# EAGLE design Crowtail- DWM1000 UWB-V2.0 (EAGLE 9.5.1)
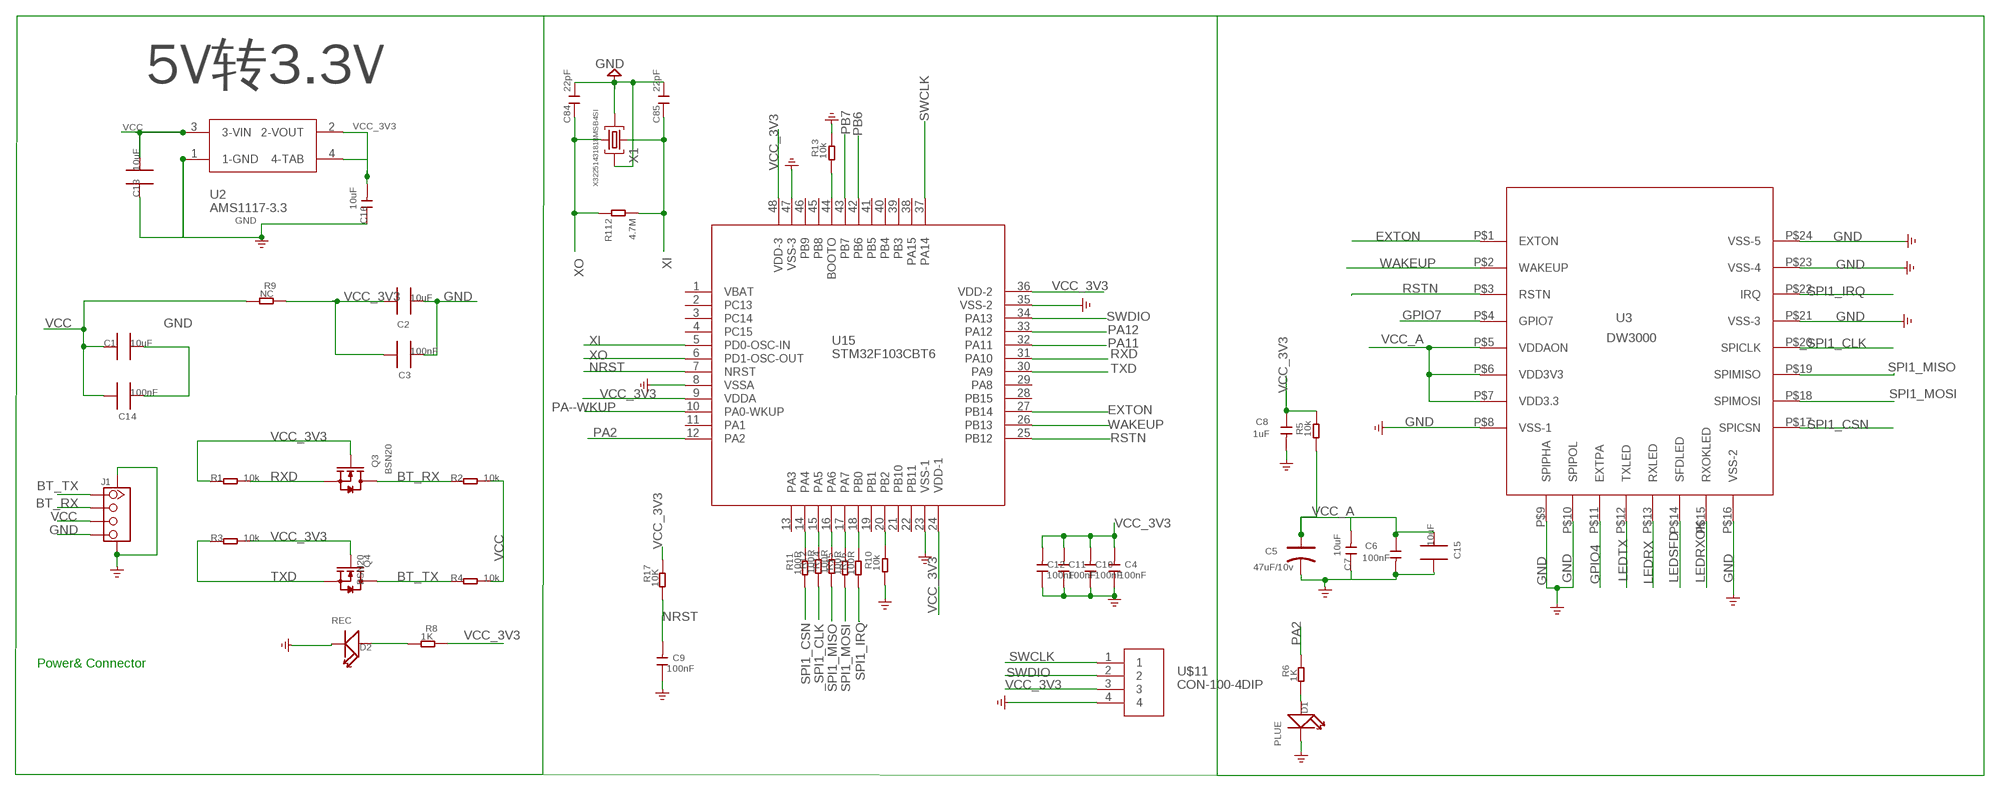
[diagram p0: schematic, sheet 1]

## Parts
C1  10uF  C0805_S  [0805_S]
C2  10uF  C0805_S  [0805_S]
C3  100nF  C0603_S  [0603_S]
C4  100nF  C-0603  [C0603]
C5  47uF/10v  CAP-AVX-B  [AVX-B]
C6  100nF  C-0603  [C0603]
C7  10uF  C-0805  [C0805]
C8  1uF  C-0603  [C0603]
C9  100nF  C-0603  [C0603]
C10  100nF  C-0603  [C0603]
C11  100nF  C-0603  [C0603]
C12  100nF  C-0603  [C0603]
C13  10uF  C0805_S  [0805_S]
C14  100nF  C0603_S  [0603_S]
C15  10uF  C0805_S  [0805_S]
C16  10uF  C-0805  [C0805]
C84  22pF  C0603  [0603]
C85  22pF  C0603  [0603]
D1  PLUE  LED'0603'  [LED-0603]
D2  REC  LED'0603'  [LED-0603]
J1  TWIG-4P-2.0-SMD-FEMALE-REINFORCE'90D'  [4P-SMD-2.0-90D]
Q3  BSN20  MOSFET-N'SOT23'  [SOT23]
Q4  BSN20  MOSFET-N'SOT23'  [SOT23]
R1  10k  R-0603  [R0603]
R2  10k  R-0603  [R0603]
R3  10k  R-0603  [R0603]
R4  10k  R-0603  [R0603]
R5  10k  R-0603  [R0603]
R6  1K  R-0603  [R0603]
R8  1K  R-0603  [R0603]
R9  NC  R-0603  [R0603]
R10  10k  R-0603  [R0603]
R11  100R  R-0603  [R0603]
R12  100R  R-0603  [R0603]
R13  10k  R-0603  [R0603]
R14  100R  R-0603  [R0603]
R15  100R  R-0603  [R0603]
R16  100R  R-0603  [R0603]
R17  10K  R-0603  [R0603]
R112  4.7M  R0603  [R0603]
U2  AMS1117-3.3  [AMS1117-3.3-SOT223]
U3  DW3000  DW1000  [DW1000]
U15  STM32F103CBT6  [LQFO48]
U$11  CON-100-4DIP  [DIP-2.54-4]
X1  X32251431818MSB4SI  CRYSTAL-3.2-2.5  [CRYSTAL-3.2-2.5]

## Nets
_SPI1_CLK: R12.1 U3.P$20(SPICLK)
BT_RX: J1.2 Q3.3(D) R2.1
BT_TX: J1.1 Q4.3(D) R4.1
EXTON: U3.P$1(EXTON) U15.27(PB14)
GND: C1.2 C2.2 C3.2 C4.1 C5.- C6.2 C7.1 C8.2 C9.1 C10.1 C11.1 C12.1 C13.1 C14.2 C15.1 C16.1 C84.1 C85.1 D1.- D2.- J1.4 J1.SS1 J1.SS2 R10.1 R13.2 U2.1(1-GND) U3.P$8(VSS-1) U3.P$9(SPIPHA) U3.P$10(SPIPOL) U3.P$16(VSS-2) U3.P$21(VSS-3) U3.P$23(VSS-4) U3.P$24(VSS-5) U15.8(VSSA) U15.23(VSS-1) U15.35(VSS-2) U15.47(VSS-3) U$11.4 X1.2(GND) X1.4(GND)
GPIO4: U3.P$11(EXTPA)
GPIO7: U3.P$4(GPIO7)
LEDRX: U3.P$13(RXLED)
LEDRXOK: U3.P$15(RXOKLED)
LEDSFD: U3.P$14(SFDLED)
LEDTX: U3.P$12(TXLED)
N$2: R10.2 U15.20(PB2)
N$3: R13.1 U15.44(BOOTO)
N$4: D1.+ R6.1
N$5: D2.+ R8.1
N$7: R11.2 U15.14(PA4)
N$8: R12.2 U15.15(PA5)
N$9: R14.2 U15.16(PA6)
N$10: R15.2 U15.17(PA7)
N$12: R16.2 U15.18(PB0)
NRST: C9.2 R17.1 U15.7(NRST)
PA2: R6.2 U15.12(PA2)
PA11: U15.32(PA11)
PA12: U15.33(PA12)
PA--WKUP: U15.10(PA0-WKUP)
PB6: U15.42(PB6)
PB7: U15.43(PB7)
RSTN: U3.P$3(RSTN) U15.25(PB12)
RXD: Q3.2(S) R1.2 U15.31(PA10)
SPI1_CSN: R11.1 U3.P$17(SPICSN)
SPI1_IRQ: R16.1 U3.P$22(IRQ)
SPI1_MISO: R14.1 U3.P$19(SPIMISO)
SPI1_MOSI: R15.1 U3.P$18(SPIMOSI)
SWCLK: U15.37(PA14) U$11.1
SWDIO: U15.34(PA13) U$11.2
TXD: Q4.2(S) R3.1 U15.30(PA9)
VCC: C1.1 C13.2 C14.1 J1.3 R2.2 R4.2 R9.1 U2.3(3-VIN)
VCC_3V3: C2.1 C3.1 C4.2 C8.1 C10.2 C11.2 C12.2 C16.2 Q3.1(G) Q4.1(G) R1.1 R3.2 R5.2 R8.2 R9.2 R17.2 U2.2(2-VOUT) U2.4(4-TAB) U15.9(VDDA) U15.24(VDD-1) U15.36(VDD-2) U15.48(VDD-3) U$11.3
VCC_A: C5.+ C6.1 C7.2 C15.2 R5.1 U3.P$5(VDDAON) U3.P$6(VDD3V3) U3.P$7(VDD3.3)
WAKEUP: U3.P$2(WAKEUP) U15.26(PB13)
XI: C85.2 R112.1 U15.5(PD0-OSC-IN) X1.3(C2)
XO: C84.2 R112.2 U15.6(PD1-OSC-OUT) X1.1(C1)
Unconnected: U15.1(VBAT) U15.2(PC13) U15.3(PC14) U15.4(PC15) U15.11(PA1) U15.13(PA3) U15.19(PB1) U15.21(PB10) U15.22(PB11) U15.28(PB15) U15.29(PA8) U15.38(PA15) U15.39(PB3) U15.40(PB4) U15.41(PB5) U15.45(PB8) U15.46(PB9)

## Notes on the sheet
- 5V转3.3V
- Power& Connector

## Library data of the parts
C1 C2 C13 C15 = CPT_SMD:C0805
C3 C14 = CPT_SMD:C0603
C4 C6 C8-C12 = discrete:C*: Ceramic Capacitors
C5 = discrete:CAP*: Electrolytic Capacitors,Tantalum Capacitors and Super Capacitors
C7 C16 = Discrete:C*: Ceramic Capacitors
C84 C85 = cooper:C0603
D1 D2 = discrete:LED*
J1 = Connector:TWIG-4P-2.0-SMD-FEMALE-REINFORCE
Q3 Q4 = discrete:MOSFET-N: IRLL014: http://www.vishay.com/docs/91319/sihll014.pdf
R1-R6 R8-R17 = discrete:R*
R112 = cooper:R0603
U2 = Crowtail- LoRA module-V1.0:AMS1117-3.3
U3 = DW1000:DW1000
U15 = DFN8:STM32F103CBT6
U$11 = DW1000:CON-100-4DIP
X1 = SmartPrj:CRYSTAL-3.2-2.5

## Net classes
0 default: width 0.152 mm, drill 0.305 mm, clearance 0.203 mm

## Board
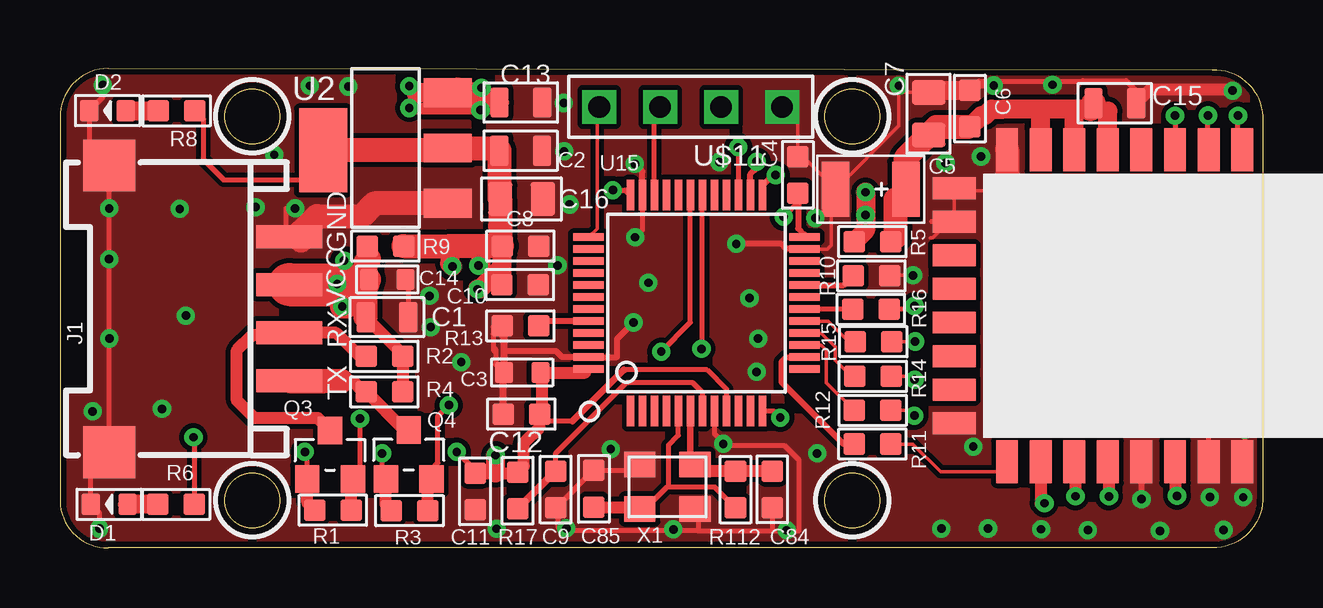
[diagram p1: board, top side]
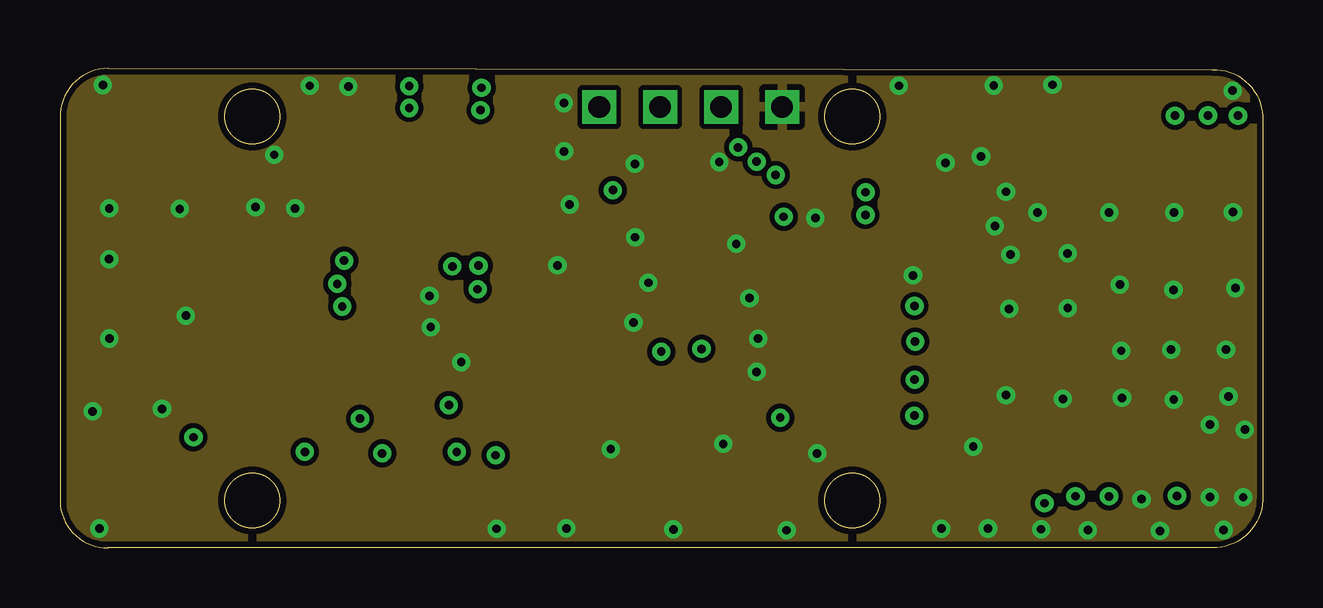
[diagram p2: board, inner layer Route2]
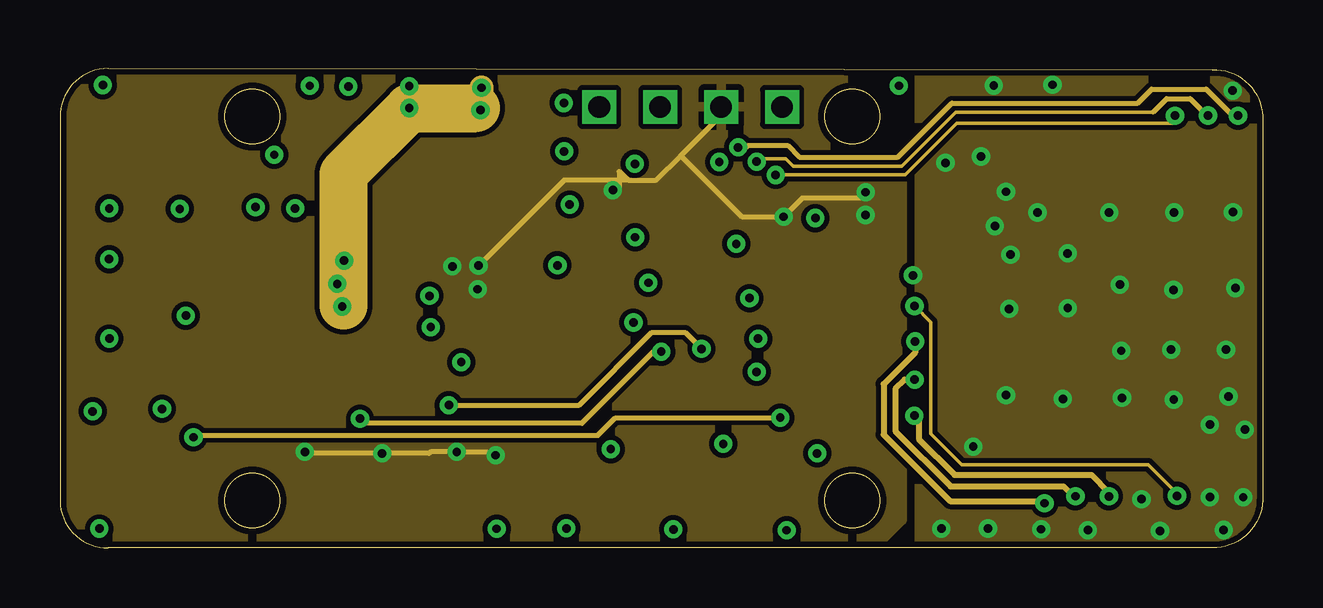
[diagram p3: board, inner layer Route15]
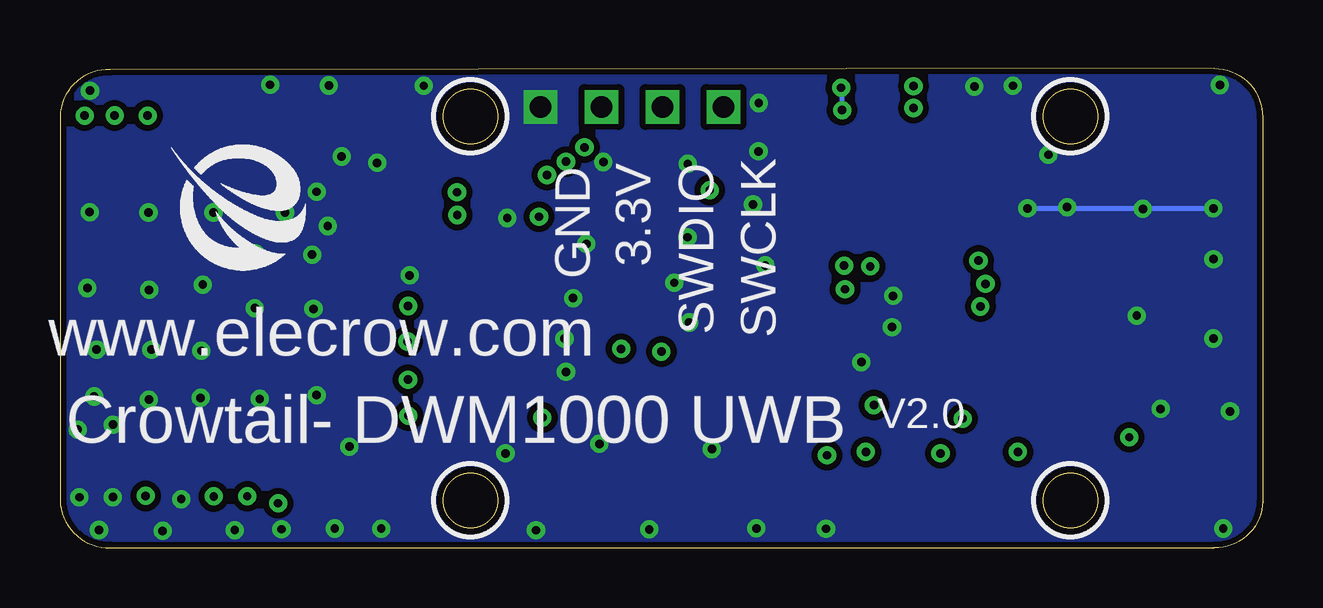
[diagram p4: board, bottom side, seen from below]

Size 50.11 x 19.97 mm. Coordinates in mm from the lower left corner, seen from the top.
Outline: 2.01,19.97 48.01,19.92 arc-90 50.11,17.97 50.11,1.97 arc-90 48.01,0 2.01,0 arc-90 0,1.93 0,17.93 arc-90 2.01,19.97
Outline: circle at 8.01,17.97 radius 1.14
Outline: circle at 8.01,1.97 radius 1.14
Outline: circle at 33.01,1.97 radius 1.14
Outline: circle at 33.01,17.97 radius 1.14
Copper layers (1+2*15+16): Top 0.035mm / dielectric 1.5mm / Route2 0.035mm / dielectric 0.15mm / Route15 0.035mm / dielectric 0.2mm / Bottom 0.035mm
Design rules "default *": minimum track width 6mil, minimum drill 0.3mm, track to track 6mil, track to pad 5mil, pad to pad 5mil, via to via 6mil, smd to smd 6mil, copper to edge 10mil, drill to drill 6mil, minimum pad ring 10mil, minimum via ring 8mil, stop-mask expansion 4mil, vias tented up to drill 30mil, thermal gap 10mil

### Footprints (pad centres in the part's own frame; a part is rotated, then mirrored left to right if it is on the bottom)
0805_S = smd 0.762 x 1.27: 1 -0.889,0; 2 0.889,0
0603_S = smd 0.762 x 0.889: 1 -0.762,0; 2 0.762,0
C0603 = smd 0.889 x 0.889: 1 -0.762,0; 2 0.762,0
AVX-B = smd 1.143 x 2.286: + -1.46,0; - 1.46,0
C0805 = smd 1.016 x 1.397: 1 -0.889,0; 2 0.889,0
0603 = smd 0.889 x 0.889: 1 -0.762,0; 2 0.762,0
LED-0603 = smd 0.762 x 0.889: + -0.762,0; - 0.762,0
4P-SMD-2.0-90D = smd 0.965 x 2.74: 1 -3,-0.1; 2 -1,-0.1; 3 1,-0.1; 4 3,-0.1 | smd 2.159 x 2.184: SS1 -5.974,7.4; SS2 5.974,7.4
SOT23 = smd 1.016 x 1.143: 1 -0.95,-1.016; 2 0.95,-1.016; 3 0,1.016
R0603 = smd 0.889 x 0.889: 1 -0.762,0; 2 0.762,0
AMS1117-3.3-SOT223 = smd 1.2 x 2: 1 -2.2,-2.7; 2 0.1,-2.7; 3 2.4,-2.7 | smd 3.5 x 2: 4 0,2.5
DW1000 = smd 1.778 x 0.914: P$1 -6.5,9.8; P$2 -6.5,8.4; P$3 -6.5,7; P$4 -6.5,5.6; P$5 -6.5,4.2; P$6 -6.5,2.8; P$7 -6.5,1.4; P$8 -6.5,0; P$17 6.5,0; P$18 6.5,1.4; P$19 6.5,2.8; P$20 6.5,4.2; P$21 6.5,5.6; P$22 6.5,7; P$23 6.5,8.4; P$24 6.5,9.8 | smd 0.914 x 1.778: P$9 -3.5,-2.2; P$10 -4.9,-2.2; P$11 -2.1,-2.2; P$12 -0.7,-2.2; P$13 0.7,-2.2; P$14 2.1,-2.2; P$15 3.5,-2.2; P$16 4.9,-2.2
LQFO48 = smd 1.27 x 0.3: 1 -4.5,2.75; 2 -4.5,2.25; 3 -4.5,1.75; 4 -4.5,1.25; 5 -4.5,0.75; 6 -4.5,0.25; 7 -4.5,-0.25; 8 -4.5,-0.75; 9 -4.5,-1.25; 10 -4.5,-1.75; 11 -4.5,-2.25; 12 -4.5,-2.75; 25 4.5,-2.75; 26 4.5,-2.25; 27 4.5,-1.75; 28 4.5,-1.25; 29 4.5,-0.75; 30 4.5,-0.25; 31 4.5,0.25; 32 4.5,0.75; 33 4.5,1.25; 34 4.5,1.75; 35 4.5,2.25; 36 4.5,2.75 | smd 0.3 x 1.27: 13 -2.75,-4.5; 14 -2.25,-4.5; 15 -1.75,-4.5; 16 -1.25,-4.5; 17 -0.75,-4.5; 18 -0.25,-4.5; 19 0.25,-4.5; 20 0.75,-4.5; 21 1.25,-4.5; 22 1.75,-4.5; 23 2.25,-4.5; 24 2.75,-4.5; 37 2.75,4.5; 38 2.25,4.5; 39 1.75,4.5; 40 1.25,4.5; 41 0.75,4.5; 42 0.25,4.5; 43 -0.25,4.5; 44 -0.75,4.5; 45 -1.25,4.5; 46 -1.75,4.5; 47 -2.25,4.5; 48 -2.75,4.5
DIP-2.54-4 = drill 0.9 square: 1 0,0; 2 2.54,0; 3 5.08,0; 4 7.62,0
CRYSTAL-3.2-2.5 = smd 1.3 x 1.05: 1 -1.15,-0.925; 2 1.15,-0.925; 3 1.15,0.925; 4 -1.15,0.925

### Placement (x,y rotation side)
C1  13.62,9.61 0 top
C2  19.19,16.54 0 top
C3  19.26,7.3 180 top
C4  30.75,15.53 270 top
C5  33.78,14.94 180 top
C6  37.91,18.29 90 top
C7  36.19,18.08 270 top
C8  19.18,12.56 0 top
C9  20.65,2.41 90 top
C10  19.16,10.96 180 top
C11  17.29,2.34 90 top
C12  19.23,5.57 0 top
C13  19.2,18.55 180 top
C14  13.64,11.17 0 top
C15  43.95,18.52 180 top
C16  19.23,14.53 180 top
C84  29.68,2.42 90 top
C85  22.25,2.45 270 top
D1  2.05,1.81 180 top
D2  1.98,18.21 180 top
J1  9.45,9.95 90 top
Q3  11.25,3.87 0 top
Q4  14.53,3.88 0 top
R1  11.37,1.56 0 top
R2  13.52,7.97 0 top
R3  14.56,1.55 180 top
R4  13.52,6.49 0 top
R5  33.85,12.75 180 top
R6  4.84,1.8 0 top
R8  4.86,18.2 0 top
R9  13.56,12.57 0 top
R10  33.8,11.33 180 top
R11  33.85,4.32 180 top
R12  33.86,5.72 180 top
R13  19.18,9.24 180 top
R14  33.87,7.14 180 top
R15  33.89,8.59 180 top
R16  33.79,9.93 180 top
R17  19.07,2.37 90 top
R112  28.15,2.42 90 top
U2  13.46,16.55 90 top
U3  39.46,10.08 270 top
U15  26.52,10.19 90 top
U$11  22.47,18.36 0 top
U$15  [LOGO]  42.13,15.3 0 bottom
X1  25.31,2.54 180 top

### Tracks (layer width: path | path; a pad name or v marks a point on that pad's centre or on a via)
_SPI1_CLK  (via drill 0.35)
  Top 0.152: 43.71,3.53 U3.P$20 | v35.6,5.5 35.38,5.72 R12.1 | v43.71,2.14
  Top 0.203: U3.P$20
  Top 0.5: v43.71,2.14 43.71,3.53
  Route15 0.25: v35.6,5.5 35.79,5.31 35.79,4.52 37.28,3.03 42.98,3.03 43.71,2.3 v43.71,2.14
BT_RX
  Top 0.25: R2.1 12.49,7.97 | J1.2 9.46,8.86
  Top 0.5: Q3.3 10.75,5.39 8.11,5.39 7.37,6.13 7.37,8.22 8.01,8.86 9.46,8.86 | J1.2 11.51,8.95 12.49,7.97
BT_TX
  Top 0.152: Q4.3 14.42,4.9 14.23,4.9 12.62,6.5 12.19,6.93 11.72,6.93 | 11.03,6.93 12.31,6.93 R4.1
  Top 0.203: 9.57,6.93 J1.1
  Top 0.25: J1.1 12.18,6.95 | 14.35,4.9 14.42,4.9
  Top 0.5: 12.18,6.95 12.62,6.5 | R4.1 14.35,4.9
  Top 1: 11.72,6.93 11.03,6.93 9.57,6.93
EXTON  (via drill 0.35)
  Top 0.2: v28.26,16.68 28.27,16.67 U15.27 | U3.P$1 49.08,16.76 v49.08,18
  Route15 0.2: v28.26,16.68 28.59,16.68 28.67,16.76 30.32,16.76 30.81,16.27 34.92,16.27 37.17,18.52 44.91,18.52 45.49,19.11 47.76,19.11 48.86,18 v49.08,18
GND  (via drill 0.35)
  Top 0.152: 24.27,13.24 v23.97,12.93 | 36.25,12.92 36.37,12.92 37.03,13.58 | U3.P$9 U3.P$10 37.37,14.87 39.46,14.87 | U$11.4 30.75,17.7 C4.1 30.97,16.29 C5.- 34.95,17.57 34.95,19.12 | 34.95,19.12 v34.95,19.25 | C7.1 35.1,18.97 34.95,19.12 | U15.23 31.96,12.44 32.13,12.61 32.13,14 32.02,14.11 32.02,14.58 32.35,14.91 | R10.1 34.59,11.35 v35.54,11.35
  Top 0.2: v38.91,19.25 38.11,19.25 C6.2 38.3,19.44 42.59,19.44 42.61,19.46 44.42,19.46 45.1,18.78 | C14.2 14.51,11.06 C1.2 | 32.35,14.91 C5.- | 2.05,4.04 1.28,3.27 D1.- 1.64,1.45 v1.64,0.79 | J1.SS2 1.61,15.92 1.21,16.33 1.22,16.34 D2.- 1.79,18.77 v1.79,19.27 | U15.35 24.27,13.24
  Top 0.203: 10.05,12.79 9.71,12.79 J1.4 9.43,13.08 9.43,14.14 v9.8,14.14 | X1.2 23.91,3.21 C85.1 22.22,3.21 20.75,1.75 | X1.4 26.6,1.47 26.6,0.7 | 26.6,0.7 29.69,0.7 | 29.69,0.7 C84.1 | C3.2 18.15,7.64 18.15,8.27 18.08,8.19 18.08,8.9 18.08,9.2 | U3.P$24 49.37,3.69 v49.37,4.92 48.9,5.39 47.98,5.39 47.86,5.27 U3.P$23 48,3.44 | U15.8 27.27,4.76 27.77,4.26 30.18,4.26 30.78,3.65 30.78,0.7 | 29.69,0.7 30.78,0.7 | 30.78,0.7 | C9.1 20.75,1.75 | 26.6,0.7 20.91,0.7 20.75,0.85 20.75,1.75 | J1.SS1 2.05,4.04 v2.05,14.14 J1.SS2 | 37.13,5.05 U3.P$16 | 48.81,19.11 48.87,19.05 v48.86,19.04 | U3.P$9 37.03,13.58 36.32,13.58
  Top 0.25: U3.P$21 v45.06,2.02 | v45.06,2.02 | v23.89,9.38 23.2,8.69 23.2,7.94 U15.47 20.92,7.94 20.67,8.19 18.51,8.19 18.5,8.18 | U15.35 24.27,15.68 v23.96,15.99 | U15.23 31,12.46 30.25,12.46 30.05,12.66 v28.18,12.66
  Top 0.3: C12.1 18.46,7.26 C3.2 18.5,8.18 18.5,8.78 18.08,9.2 | 18.08,8.9 R13.2
  Top 0.5: C15.1 45.1,18.78 45.43,19.11 48.81,19.11
  Top 0.8: C7.1 36.28,19.05 C6.2
  Top 1: U3.P$8 39.46,14.87 v39.42,14.83 | U2.1 13.1,14.35 12.57,13.82 10.7,13.82 10.05,13.17 10.05,12.79
  Bottom 0.203: v9.8,14.14 v2.05,14.14
  other vias: 49.3,2.1 43.71,13.96 8.93,16.37 10.41,19.25 40.73,13.97 46.42,13.96 48.49,0.73 47.91,2.1 30.27,0.72 25.56,0.76 21.1,0.8 18.19,0.79 1.36,5.68 4.25,5.78 42.83,0.73 2.05,8.72 2.05,12.02 4.99,14.12 8.15,14.19 12.01,19.21 16.72,7.73 31.47,13.73 29.03,7.32 45.84,0.7 28.73,10.4 29.09,8.71 22.95,4.1 44.16,10.96 48.97,10.82 38.38,16.3 36.9,16.03 39.42,6.35 44.22,8.2 44.25,6.24 47.91,5.12 5.25,9.67 27.64,4.32 41.99,9.98 27.47,16.07 36.72,0.79 38.66,0.8 40.88,0.77 31.55,3.93 41.79,6.2 46.41,6.17 48.69,6.3 48.59,8.25 46.3,8.25 46.4,10.74 39.55,9.95 39.61,12.21 41.99,12.26 48.88,13.98 41.36,19.29 24.52,11.04 15.4,10.49 15.45,9.19 20.73,11.76 21.24,14.3 21.01,16.51 21,18.53 38.05,4.21 38.95,13.4
  pour Top (no thermals): -1.27,20.25 61,20.25 61,-0.57 -1.27,-0.57
  pour Bottom (isolate 0.254, no thermals): -0.5,20.25 61,20.25 61,-0.72 -0.5,-0.72
  pour Route2: -1.96,20.91 -1.96,-1.37 -1.81,-1.52 -1.33,-2 50.82,-2 50.82,20.8 50.46,21.16 -1.77,21.16 -1.88,21.05
  pour Route15: 35.81,20.83 35.81,-0.44 35.78,-0.47 50.73,-0.47 50.8,-0.54 50.8,19.19 49.67,20.32 49.27,20.72 35.92,20.72 35.92,20.69
N$2
  Top 0.25: U15.20 32.66,10.94 R10.2
N$3
  Top 0.203: 20.14,9.44 R13.1
  Top 0.25: U15.44 20.14,9.44
N$4
  Top 0.2: R6.1
  Top 0.8: R6.1 D1.+
N$5
  Top 0.2: 4.09,18.21 R8.1
  Top 0.8: D2.+ 4.09,18.21
N$7
  Top 0.25: U15.14 31,7.92 30.25,7.92 30.06,7.73 30.06,6.91 32.65,4.32 R11.2
N$8
  Top 0.152: U15.15 31.72,8.44 31.94,8.23 31.94,6.88 R12.2
N$9
  Top 0.152: U15.16 31.73,8.94 32.3,8.36 32.3,7.8 32.97,7.14 R14.2
N$10
  Top 0.152: R15.2 32.86,8.59 32.01,9.44 U15.17
N$12
  Top 0.2: R16.2 33.02,9.94 U15.18
NRST
  Top 0.203: 20.63,3.18 C9.2 20.65,3.93 23.61,6.89 26.35,6.89 26.77,6.46 U15.7
  Top 0.32: R17.1 20.63,3.18
PA2  (via drill 0.35)
  Top 0.2: v5.56,4.6 5.6,4.55 R6.2 | v30.01,5.42 29.74,5.69 U15.12
  Route15 0.2: v5.56,4.6 5.64,4.68 22.41,4.68 23.14,5.41 v30,5.41 v30.01,5.42
RSTN  (via drill 0.35)
  Top 0.152: U15.25 29.27,15.09 | 29.77,15.58 v29.82,15.53
  Top 0.2: v46.46,18 U3.P$3
  Top 0.24: 29.27,15.09 29.77,15.58
  Route15 0.152: v29.82,15.53 35.21,15.53 37.36,17.68 46.46,17.68 v46.46,18
RXD  (via drill 0.35)
  Top 0.2: 12.14,2.79 Q3.2 12.5,3.15 v12.5,5.37
  Top 0.203: U15.31 26.27,9.38 v25.05,8.17
  Top 0.5: R1.2 12.14,2.79
  Route15 0.2: v25.05,8.17 24.73,8.17 21.74,5.18 12.7,5.18 v12.5,5.37
SPI1_CSN
  Top 0.152: R11.1 35.54,4.32 36.7,3.16 39.38,3.16 39.41,3.14
  Top 0.203: U3.P$17 39.41,3.53 39.41,3.14
SPI1_IRQ  (via drill 0.35)
  Top 0.152: 46.46,2.2 46.52,2.14 v46.54,2.16
  Top 0.2: v35.61,10.07 35.46,9.93 R16.1
  Top 0.5: U3.P$22 46.46,2.2
  Route15 0.152: v46.54,2.16 46.54,2.26 45.34,3.46 37.57,3.46 36.29,4.74 36.29,9.38 v35.61,10.07
SPI1_MISO  (via drill 0.35)
  Top 0.152: U3.P$19 42.31,3.53 | v35.61,7 35.47,7.14 R14.1
  Top 0.5: 42.31,3.53 v42.31,2.14
  Route15 0.152: 42.27,2.1 v42.31,2.14
  Route15 0.25: v35.61,7 35.19,7 34.81,6.62 34.81,4.86 37.11,2.55 41.81,2.55 42.27,2.1
SPI1_MOSI  (via drill 0.35)
  Top 0.152: 40.86,1.85 v41.02,1.85 | v35.63,8.59 R15.1
  Top 0.5: U3.P$18 40.86,1.85
  Route15 0.152: 40.93,1.94 v41.02,1.85
  Route15 0.25: v35.63,8.59 35.63,8.13 34.32,6.82 34.32,4.71 37.09,1.94 40.93,1.94
SWCLK
  Top 0.152: U15.37 22.38,13.3 22.38,18.27 U$11.1
SWDIO
  Top 0.2: U15.34 24.77,18.12 U$11.2
TXD  (via drill 0.35)
  Top 0.2: 15.32,2.71 Q4.2 15.48,3.27 15.74,3.53 15.74,5.48 v16.2,5.94
  Top 0.203: v26.73,8.28 26.77,8.32 U15.30
  Top 0.5: R3.1 15.32,2.71
  Route15 0.2: v16.2,5.94 21.63,5.94 24.66,8.97 26.05,8.97 v26.73,8.28
VCC  (via drill 0.35)
  Top 0.152: C1.1 12.74,10.91 | J1.3 11.65,10.95 12.69,10.95 12.74,10.91 | 12.74,10.91 12.81,10.84 12.81,10.96 12.81,11.1 C14.1 12.88,12.03 | R2.2 14.19,8.06 14.19,8.16 | R4.2
  Top 0.2: 16.56,19.19 v17.52,18.23
  Top 0.25: U2.3 17.35,18.95 v17.57,19.16 | 14.83,18.95 v14.55,19.23 | 18.08,18.32 C13.2 | 11.65,10.89 11.65,10.95 | 11.65,10.89 v11.55,10.99 11.55,10.26 v11.76,10.05 11.65,10.16 11.65,10.89 | R9.1 12.79,11.95 12.74,11.89
  Top 0.5: R2.2 R4.2 | 14.19,8.16 C1.1 | v14.55,18.32 18.08,18.32
  Top 0.8: C13.2 16.56,19.19 | U2.3 14.83,18.95
  Top 1: J1.3 | 12.81,10.96 11.85,10.96 | C1.1 12.74,11.89 12.88,12.03 | C14.1 11.92,10.22 11.92,10.05 v11.76,10.05
  Top 1.8: J1.3 11.85,10.96
  Route15 0.25: 17.34,18.32 17.57,18.09 | 11.81,10.1 v11.76,10.05 | v11.84,11.96 11.84,11.28 v11.55,10.99
  Route15 1: 17.57,18.09 v17.57,19.16
  Route15 2: 17.34,18.32 v14.55,18.32 11.81,15.58 11.81,10.1
  Bottom 0.2: v17.57,19.16 17.55,19.14 17.55,18.25 v17.52,18.23
VCC_3V3  (via drill 0.35)
  Top 0.152: C3.1 20.1,7.3 | 21.88,7.3 U15.48
  Top 0.2: R3.2 13.58,1.76 | R1.1 10.3,1.87 | 32.88,12.96 R5.2 | 30.76,14.75 C4.2 30.75,14.38 v30.15,13.79 | v23.04,14.9 23.56,14.9 23.65,14.81 | Q3.1 10.3,3.77 10.36,3.83 v10.2,3.99 | v16.53,3.99 17.29,3.23 C11.2 | R8.2 5.97,17.85 5.97,16.18 6.82,15.33 11.07,15.33 11.1,15.36 11.1,16.41 U2.4 | 18.34,13.4 18.34,11.63 18.34,11.02 C10.2 | 21.35,5.27 20.28,5.27 C12.2 | R17.2 19.33,3.4 | 19.99,5.03 C12.2 | C12.2 20.1,5.68 | Q4.1 13.42,3.02 v13.42,3.93
  Top 0.203: C3.1 20.1,7.38 | 23.5,7.4 26.97,7.4 27.77,6.6 U15.9 | 19.04,3.1 R17.2 | 23.55,14.91 23.65,14.81 U15.36 | U15.48 21.89,7.3 | 31.02,13.04 U15.24
  Top 0.25: 30.76,14.75 30.76,13.3 31.02,13.04
  Top 0.3: 23.5,7.4 23.48,7.4 21.35,5.27
  Top 0.5: C11.2 18.15,3.1 19.04,3.1 | 21.88,7.3 20.1,7.3 20.1,5.68 | 13.58,1.76 Q4.1 | 10.3,1.87 Q3.1 | 19.33,3.4 19.33,4.37 19.99,5.03
  Top 0.8: v33.57,14.81 33.57,13.23 R5.2 | 16.23,12.57 16.23,11.84 v16.35,11.72 | 17.54,12.57 17.54,11.85 v17.44,11.75 | 18.34,13.4 18.4,13.34 C10.2 | 18.34,11.63 17.48,10.77 v17.4,10.77 | 18.15,3.1 v18.15,3.85
  Top 1: U2.4 16.06,16.55 U2.2 18.2,16.65 C2.1 18.31,14.56 C16.2 18.34,13.4 18.34,12.64 C8.1 17.54,12.57 16.23,12.57 R9.2
  Route15 0.2: v17.44,11.75 21,15.31 23.67,15.31 | 23.67,15.31 23.3,15.68 23.3,14.88 23.28,14.86 23.04,14.86 v23.04,14.9 | 23.67,15.31 24.83,15.31 25.86,16.34 | U$11.3 27.55,18.03 25.86,16.34 | 25.86,16.34 28.41,13.79 v30.15,13.79 30.92,14.56 33.57,14.56 v33.57,14.81 | v10.2,3.99 10.26,3.93 v13.42,3.93 15.38,3.93 15.44,3.99 v16.53,3.99 18.01,3.99 v18.15,3.85
  other vias: 33.56,13.86
  pour Route15: -0.14,20.69 34.81,20.69 35.1,20.4 35.1,1.14 33.53,-0.43 0.27,-0.43 -0.28,0.12 -0.35,0.19 -0.35,20.61
VCC_A
  Top 0.152: 36.15,17.15 C7.2 | 37.82,17.53 C6.1 38.71,18.33 40.93,18.33 | 40.93,18.33 42.35,18.33 | 42.35,18.33 42.98,18.33 | 42.26,18.12 42.26,18.24 42.35,18.33 | 40.86,18.11 40.86,18.26 40.93,18.33
  Top 0.2: 36.08,17.07 36.15,17.15 | R5.1 34.81,12.95 | 34.81,14.51 C5.+
  Top 0.25: C15.2 43.34,18.52 43.66,18.2
  Top 0.8: C6.1 38.39,18 38.54,18 38.81,18.27 39.31,18.27 39.32,18.28 42.93,18.28 | U3.P$5 43.66,18.2 | U3.P$6 42.26,18.12 | U3.P$7 40.86,18.11
  Top 1: C5.+ 35.24,16.24 36.08,17.07 | C7.2 36.53,17.53 37.82,17.53 | 34.81,14.51 34.81,12.95 | C15.2 43.06,18.41 42.98,18.33 42.93,18.28
WAKEUP  (via drill 0.35)
  Top 0.152: 29.03,15.81 v29.03,16.08
  Top 0.2: U3.P$2 47.83,16.61 v47.83,18.01
  Top 0.24: U15.26 28.77,15.56 29.03,15.81
  Route15 0.152: v29.03,16.08 29.14,16.2 30.24,16.2 30.54,15.89 35.07,15.89 37.32,18.14 45.55,18.14 | v47.83,18.01 47.78,18.01
  Route15 0.2: 47.78,18.01 47.09,18.7 46.11,18.7 45.55,18.14
XI
  Top 0.203: 24.08,1.69 X1.3 24.43,1.88 24.65,1.88 25.29,2.52 25.35,2.52 | R112.1 27.28,2.52 25.35,2.52 | 25.35,2.52 25.34,2.53 25.34,4.25 25.77,4.68 U15.5
  Top 0.5: C85.2 24.08,1.69
XO
  Top 0.203: C84.2 | 26.74,3.18 X1.1 26.27,3.65
  Top 0.28: U15.6 26.27,3.65
  Top 0.5: C84.2 R112.2 26.74,3.18

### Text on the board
tPlace: GND | VCC | RX | TX
bPlace: SWCLK | SWDIO | GND | 3.3V | www.elecrow.com | V2.0 | Crowtail- DWM1000 UWB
